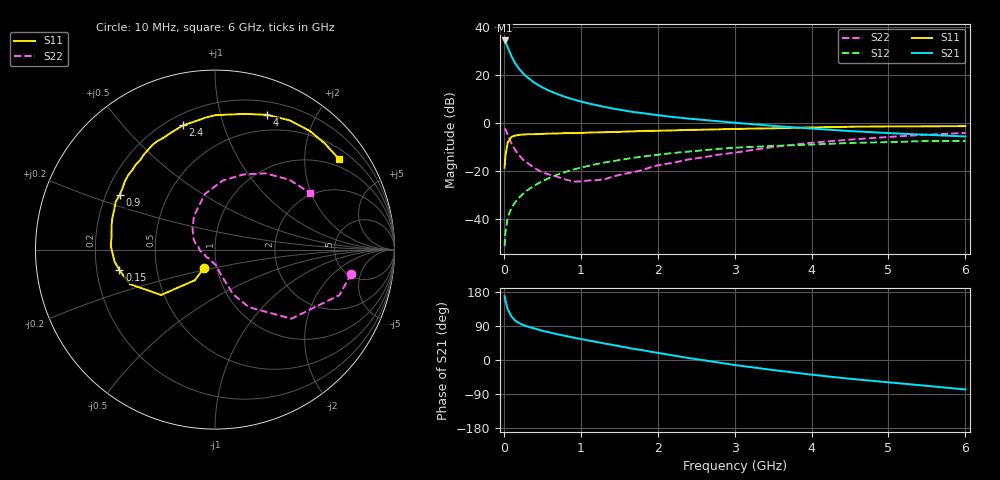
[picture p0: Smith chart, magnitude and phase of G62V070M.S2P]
! SIEMENS Small Signal Semiconductors
! BFG193
! Si NPN RF Bipolar Junction Transistor in SOT223
! VCE = 2 V  IC = 70 mA
! Common Emitter S-Parameters:  August  1996
# GHz  S  MA  R  50
!  f  S11  S21  S12  S22
! GHz  MAG  ANG  MAG  ANG  MAG  ANG  MAG  ANG
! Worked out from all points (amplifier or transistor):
!   36 points, 10 MHz to 6 GHz, reference 50 ohm
!   highest |S21| = 34.4 dB at 10 MHz (marker M1)
!   |S21| within 3 dB of that: start of sweep to 52.87 MHz
!   unconditionally stable (mu >= 1): start of sweep to 16.02 MHz; 216.8 MHz to 2.791 GHz
!   at 250 MHz: K = 1.03, MAG = 24.0 dB, |S12| = -29.6 dB
!   at 1.4 GHz: K = 1.09, MAG = 9.2 dB, |S12| = -16.0 dB
!   at 6 GHz: K = 0.98, MSG = 0.9 dB, |S12| = -7.5 dB
!   S11 on the Smith chart (normalised r, x): 10 MHz: 0.87, -0.18; 150 MHz: 0.30, -0.10; 900 MHz: 0.26, +0.25; 2.4 GHz: 0.26, +0.74; 4 GHz: 0.33, +1.41; 6 GHz: 0.77, +2.88
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0.01  0.1164 -120.9  52.31 168.4  0.0027 77.3  0.7715 -10.0
0.02  0.2041 -123.3  49.31 158.2  0.0051 76.0  0.7381 -20.1
0.05  0.3925 -139.9  37.98 134.1  0.0109 65.7  0.5743 -42.1
0.1  0.5123 -158.0  24.4 114.4  0.017 63.8  0.3724 -59.5
0.15  0.5451 -167.9  17.21 103.5  0.0226 65.4  0.2685 -68.0
0.2  0.564 -173.4  13.3 97.3  0.028 68.1  0.2114 -70.4
0.25  0.5712 -177.9  10.77 92.5  0.0333 68.4  0.1707 -73.8
0.3  0.5807 178.0  9.054 88.8  0.039 69.4  0.1491 -76.3
0.4  0.5814 172.4  6.853 83.0  0.0499 69.5  0.1143 -80.3
0.5  0.5916 166.9  5.503 77.2  0.0609 68.4  0.0932 -84.1
0.6  0.5984 162.9  4.612 72.5  0.0724 67.1  0.0833 -89.2
0.7  0.6037 158.6  3.972 67.8  0.0839 65.6  0.075 -97.2
0.9  0.6125 150.1  3.1 59.4  0.1065 61.5  0.0599 -115.2
1.1  0.6292 143.1  2.549 51.5  0.1273 57.8  0.0631 -137.6
1.6  0.6622 126.6  1.77 32.6  0.1787 46.4  0.089 177.2
2.2  0.6982 109.7  1.328 12.1  0.2359 32.0  0.1475 146.3
2.4  0.7151 104.4  1.231 5.2  0.2528 27.6  0.1731 136.2
3.5  0.7731 78.0  0.868 -26.5  0.3318 -0.5  0.3151 100.2
4  0.8055 68.8  0.762 -38.7  0.354 -10.4  0.3871 83.7
4.5  0.8319 59.9  0.676 -49.6  0.382 -20.7  0.4484 69.1
5.5  0.851 43.9  0.565 -68.2  0.4203 -44.0  0.5691 43.1
6  0.8551 36.1  0.522 -77.8  0.4218 -57.3  0.6174 30.6
